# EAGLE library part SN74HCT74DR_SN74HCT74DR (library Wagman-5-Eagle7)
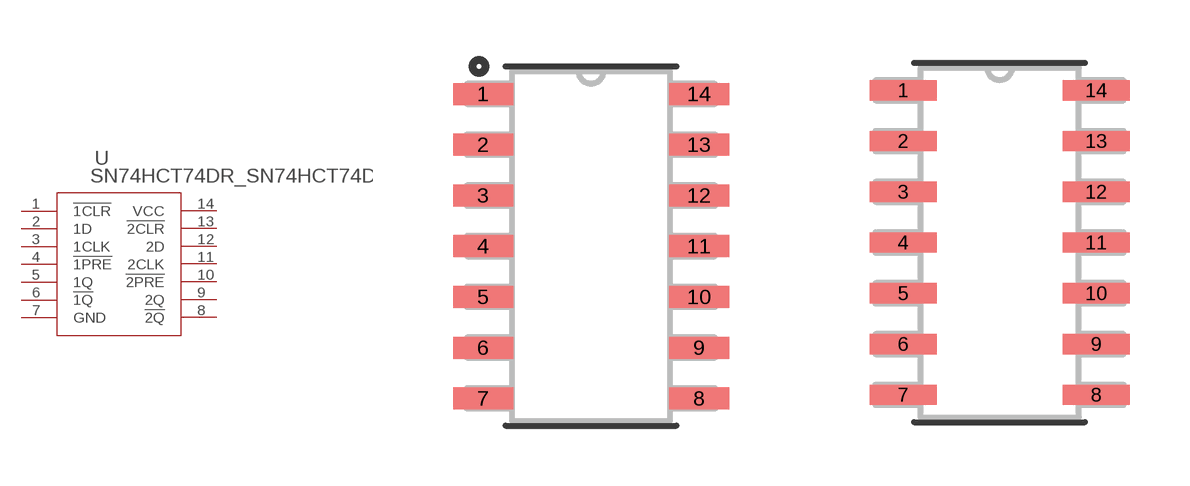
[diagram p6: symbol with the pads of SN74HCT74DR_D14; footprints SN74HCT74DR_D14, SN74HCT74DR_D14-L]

Designator prefix U

## SN74HCT74DR_SN74HCT74DR (MANUFACTURER_PART_NUMBER: SN74HCT74DR; VENDOR: Vendor)  [SN74HCT74DR_D14]
1  !1CLR  in
2  1D  in
3  1CLK  in
4  !1PRE  in
5  1Q  out
6  !1Q  out
7  GND  pwr
8  !2Q  out
9  2Q  out
10  !2PRE  in
11  2CLK  in
12  2D  in
13  !2CLR  in
14  VCC  pwr

## SN74HCT74DR_SN74HCT74DRD14-L (MANUFACTURER_PART_NUMBER: SN74HCT74DR; VENDOR: Vendor)  [SN74HCT74DR_D14-L]
Pads as for SN74HCT74DR_D14

## SN74HCT74DR_SN74HCT74DRD14-M (MANUFACTURER_PART_NUMBER: SN74HCT74DR; VENDOR: Vendor)  [SN74HCT74DR_D14-M]
Pads as for SN74HCT74DR_D14

## Footprint SN74HCT74DR_D14 (pad centres in mm)
smd 1.5 x 0.55: 1 -2.7,3.81; 2 -2.7,2.54; 3 -2.7,1.27; 4 -2.7,0; 5 -2.7,-1.27; 6 -2.7,-2.54; 7 -2.7,-3.81; 8 2.7,-3.81; 9 2.7,-2.54; 10 2.7,-1.27; 11 2.7,0; 12 2.7,1.27; 13 2.7,2.54; 14 2.7,3.81

## Footprint SN74HCT74DR_D14-L (pad centres in mm)
smd 1.676 x 0.508: 1 -2.413,3.81; 2 -2.413,2.54; 3 -2.413,1.27; 4 -2.413,0; 5 -2.413,-1.27; 6 -2.413,-2.54; 7 -2.413,-3.81; 8 2.413,-3.81; 9 2.413,-2.54; 10 2.413,-1.27; 11 2.413,0; 12 2.413,1.27; 13 2.413,2.54; 14 2.413,3.81

## Footprint SN74HCT74DR_D14-M (pad centres in mm)
smd 2.286 x 0.61: 1 -2.515,3.81; 2 -2.515,2.54; 3 -2.515,1.27; 4 -2.515,0; 5 -2.515,-1.27; 6 -2.515,-2.54; 7 -2.515,-3.81; 8 2.515,-3.81; 9 2.515,-2.54; 10 2.515,-1.27; 11 2.515,0; 12 2.515,1.27; 13 2.515,2.54; 14 2.515,3.81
